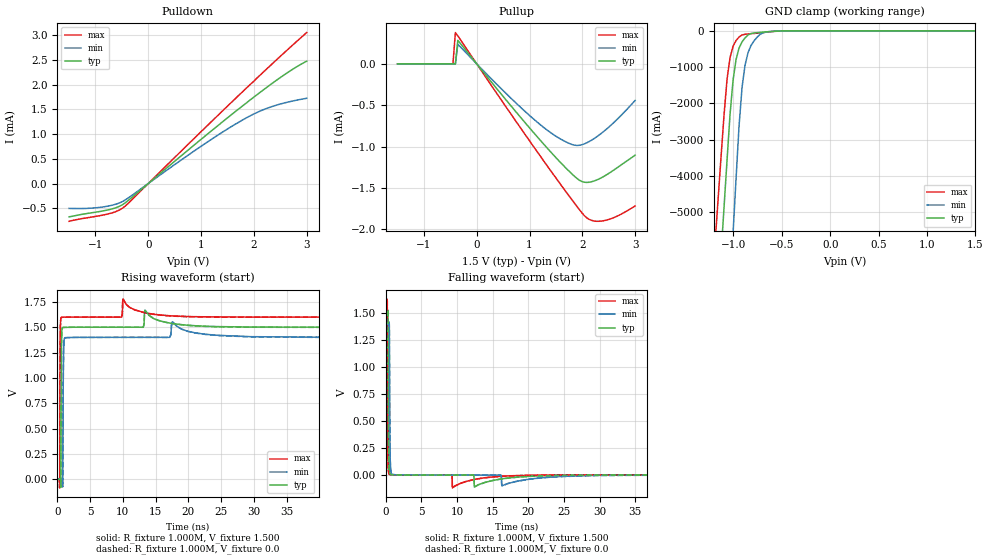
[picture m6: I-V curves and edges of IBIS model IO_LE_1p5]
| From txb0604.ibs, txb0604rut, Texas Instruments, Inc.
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|   Model IO_LE_1p5
[Model] IO_LE_1p5
Model_type 3-state
Polarity   Non-Inverting
Enable   Active-High
Vmeas =  0.750V
Cref =  15.000pF
Rref =  1.000M
Vref =  0.0V
C_comp   3.930pF   3.640pF   4.130pF
[Temperature Range]   27.000   0.125k   -40.000
[Voltage Range]   1.500V   1.400V   1.600V
[Pullup Reference]   1.500V   1.400V   1.600V
[Pulldown Reference]   0.0V   0.0V   0.0V
[POWER Clamp Reference]   1.500V   1.400V   1.600V
[GND Clamp Reference]   0.0V   0.0V   0.0V
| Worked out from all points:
|   slope of the pulldown table from 0 to 0.225 V, typ, clamps not added: 1.11 kohm
|   slope of the pullup table from 0 to 0.225 V, typ, clamps not added: 1.26 kohm
|   GND clamp passes 1 mA (typ) near -0.43 V on its own axis
|   rising waveform, R_fixture 1.000M, V_fixture 1.500: 20-80 % time 60.8ps typ, 73.5ps min, 49.8ps max; typ from 0.002 V to 1.5 V
|   rising waveform, R_fixture 1.000M, V_fixture 0.0: 20-80 % time 60.7ps typ, 73.1ps min, 49.6ps max; typ from 0 V to 1.5 V
|   falling waveform, R_fixture 1.000M, V_fixture 1.500: 20-80 % time 55.9ps typ, 72.8ps min, 48.4ps max; typ from 1.5 V to 0.002 V
|   falling waveform, R_fixture 1.000M, V_fixture 0.0: 20-80 % time 56.2ps typ, 73ps min, 48.5ps max; typ from 1.5 V to 0 V
[Pulldown]
|Voltage   I(typ)   I(min)   I(max)
-1.5V     -672.6uA   -502.3uA   -763.1uA
-1.132V   -601uA     -500.8uA   -687.9uA
-856mV    -553uA     -472.8uA   -636.9uA
-626mV    -493.6uA   -421.5uA   -571.6uA
-442mV    -394.4uA   -335.4uA   -460.3uA
984mV     878.4uA    740.7uA    1.031mA
1.444V    1.278mA    1.064mA    1.506mA
1.812V    1.59mA     1.3mA      1.881mA
2.088V    1.818mA    1.449mA    2.16mA
2.318V    2.001mA    1.546mA    2.389mA
2.686V    2.274mA    1.655mA    2.75mA
3V        2.471mA    1.722mA    3.049mA
[Pullup]
|Voltage   I(typ)   I(min)   I(max)
-1.5V     2.112nA    2.707nA    9.902nA
-450mV    108.3nA    7.187nA    723.7nA
-404mV    161.7nA    123.6nA    378.7uA
-358mV    284.8uA    236.7uA    338.3uA
608mV     -476.5uA   -390.3uA   -569.6uA
1.252V    -958.7uA   -760.2uA   -1.159mA
1.758V    -1.304mA   -964.1uA   -1.605mA
2.034V    -1.431mA   -968.6uA   -1.833mA
2.172V    -1.426mA   -923.9uA   -1.892mA
2.402V    -1.363mA   -818.9uA   -1.898mA
2.678V    -1.248mA   -659.3uA   -1.836mA
3V        -1.104mA   -442.7uA   -1.719mA
[GND_clamp]
|Voltage   I(typ)   I(min)   I(max)
-1.5V     -21.77A    -29.65A    -17.82A
-1.19V    -8.766A    -14.61A    -5.864A
-1.159V   -7.466A    -13.1A     -4.668A
-1.128V   -6.165A    -11.6A     -3.473A
-1.097V   -4.864A    -10.09A    -2.32A
-1.066V   -3.563A    -8.59A     -1.334A
-1.004V   -1.365A    -5.582A    -426.6mA
-911mV    -303.9mA   -1.56A     -113.8mA
-880mV    -195.6mA   -944.5mA   -95.38mA
-818mV    -75mA      -403.2mA   -78.97mA
-663mV    -28.8mA    -34.23mA   -37.49mA
1.5V      0A         0A         0A
[Ramp]
| variable   typ   min   max
dV/dt_r   0.899/59.226p   0.839/73.471p   0.959/48.176p
dV/dt_f   0.899/58.629p   0.839/71.453p   0.959/48.414p
R_load = 1.000M
[Rising Waveform]
R_fixture= 1.000M
V_fixture= 1.500
V_fixture_min= 1.400
V_fixture_max= 1.600
|time   V(typ)   V(min)   V(max)
0s        1.657mV    1.951mV    1.513mV
380ps     1.314mV    1.914mV    -84.08mV
450ps     4.778mV    1.808mV    1.268V
580ps     453.7mV    1.575mV    1.592V
660ps     1.373V     3.255mV    1.597V
830ps     1.496V     -63.51mV   1.598V
940ps     1.498V     1.108V     1.598V
1.1ns     1.498V     1.39V      1.599V
10.05ns   1.5V       1.4V       1.777V
120ns     1.5V       1.4V       1.6V
[Rising Waveform]
R_fixture= 1.000M
V_fixture= 0.0
V_fixture_min= 0.0
V_fixture_max= 0.0
|time   V(typ)   V(min)   V(max)
0s        723.6nV    145.4uV    -1.311uV
380ps     -345.4uV   108.6uV    -85.6mV
450ps     3.093mV    3.227uV    1.267V
580ps     452.5mV    -239.7uV   1.592V
660ps     1.373V     1.414mV    1.597V
830ps     1.496V     -65.39mV   1.598V
940ps     1.498V     1.107V     1.598V
1.09ns    1.498V     1.388V     1.599V
10.05ns   1.5V       1.4V       1.777V
120ns     1.498V     1.398V     1.598V
[Falling Waveform]
R_fixture= 1.000M
V_fixture= 1.500
V_fixture_min= 1.400
V_fixture_max= 1.600
|time   V(typ)   V(min)   V(max)
0s        1.5V       1.4V       1.6V
230ps     1.494V     1.401V     1.606V
280ps     1.483V     1.4V       432mV
330ps     1.518V     1.396V     145.2mV
450ps     127.9mV    1.386V     15.08mV
520ps     40.14mV    1.353V     6.994mV
610ps     11.69mV    268.6mV    4.491mV
790ps     4.132mV    17.63mV    2.863mV
9.37ns    32.72uV    47.21uV    -118.5mV
120ns     1.683mV    1.995mV    1.524mV
[Falling Waveform]
R_fixture= 1.000M
V_fixture= 0.0
V_fixture_min= 0.0
V_fixture_max= 0.0
|time   V(typ)   V(min)   V(max)
0s        1.498V     1.398V     1.598V
230ps     1.492V     1.398V     1.605V
280ps     1.481V     1.398V     431mV
330ps     1.516V     1.394V     144.9mV
450ps     127.6mV    1.384V     15.05mV
520ps     40.07mV    1.351V     6.964mV
610ps     11.65mV    268.1mV    4.464mV
790ps     4.101mV    17.56mV    2.836mV
9.37ns    7.589uV    20.56uV    -118.5mV
120ns     27.02uV    190.2uV    9.893uV
